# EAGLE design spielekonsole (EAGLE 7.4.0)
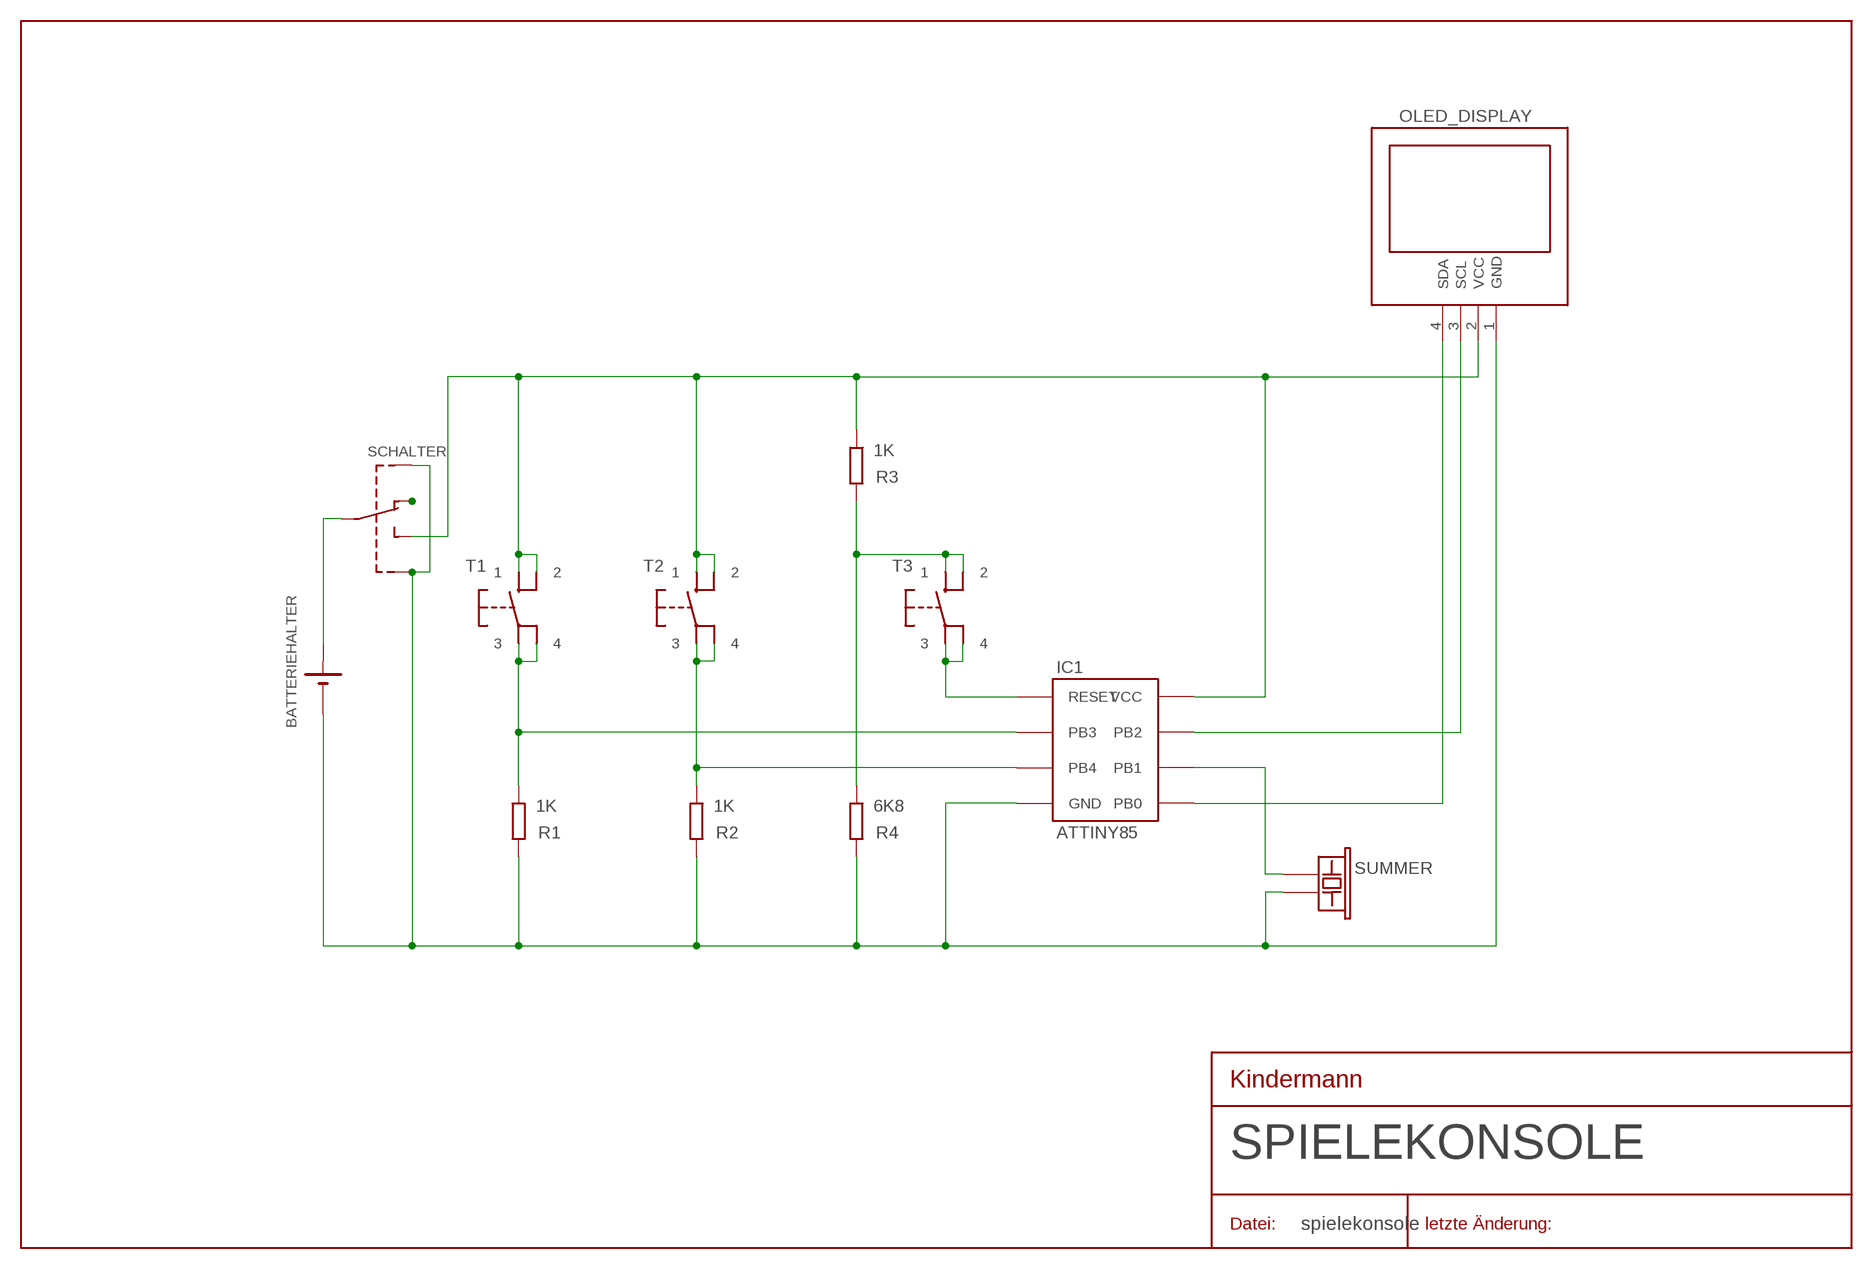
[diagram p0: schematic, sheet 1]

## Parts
BATTERIEHALTER  BATTERIEHALTER  [BATTERIEHALTER]
IC1  ATTINY85  [ATTINY85]
OLED_DISPLAY  OLED_DISPLAY  [OLED_DISPLAY]
R1  1K  WID-1K  [WID-1K]
R2  1K  WID-1K  [WID-1K]
R3  1K  WID-1K  [WID-1K]
R4  6K8  WID-6K8  [WID-6K8]
SCHALTER  S1  SCHIEBESCHALTER  [SCHIEBESCHALTER]
SUMMER  SUMMER  [SUMMER]
T1  MICROTASTER  [MICROTASTER]
T2  MICROTASTER  [MICROTASTER]
T3  MICROTASTER  [MICROTASTER]

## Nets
GND: BATTERIEHALTER.2(-) IC1.4(GND) OLED_DISPLAY.1(GND) R1.2 R2.2 R4.2 SCHALTER.4 SCHALTER.5 SUMMER.2
N$3: BATTERIEHALTER.1(+) SCHALTER.2
N$4: R3.2 R4.1 T3.1 T3.2
N$6: IC1.6(PB1) SUMMER.1
N$9: IC1.1(RESET) T3.3 T3.4
PB3: IC1.2(PB3) R1.1 T1.3 T1.4
PB4: IC1.3(PB4) R2.1 T2.3 T2.4
SCL: IC1.7(PB2) OLED_DISPLAY.3(SCL)
SDA: IC1.5(PB0) OLED_DISPLAY.4(SDA)
SW1_3: SCHALTER.3
VCC: IC1.8(VCC) OLED_DISPLAY.2(VCC) R3.1 SCHALTER.1 T1.1 T1.2 T2.1 T2.2

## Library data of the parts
BATTERIEHALTER = Spielekonsole:BATTERIEHALTER
IC1 = Spielekonsole:ATTINY85
OLED_DISPLAY = Spielekonsole:OLED_DISPLAY
R1-R3 = Spielekonsole:WID-1K
R4 = Spielekonsole:WID-6K8
SCHALTER = Spielekonsole:SCHIEBESCHALTER
SUMMER = Spielekonsole:SUMMER
T1-T3 = Spielekonsole:MICROTASTER

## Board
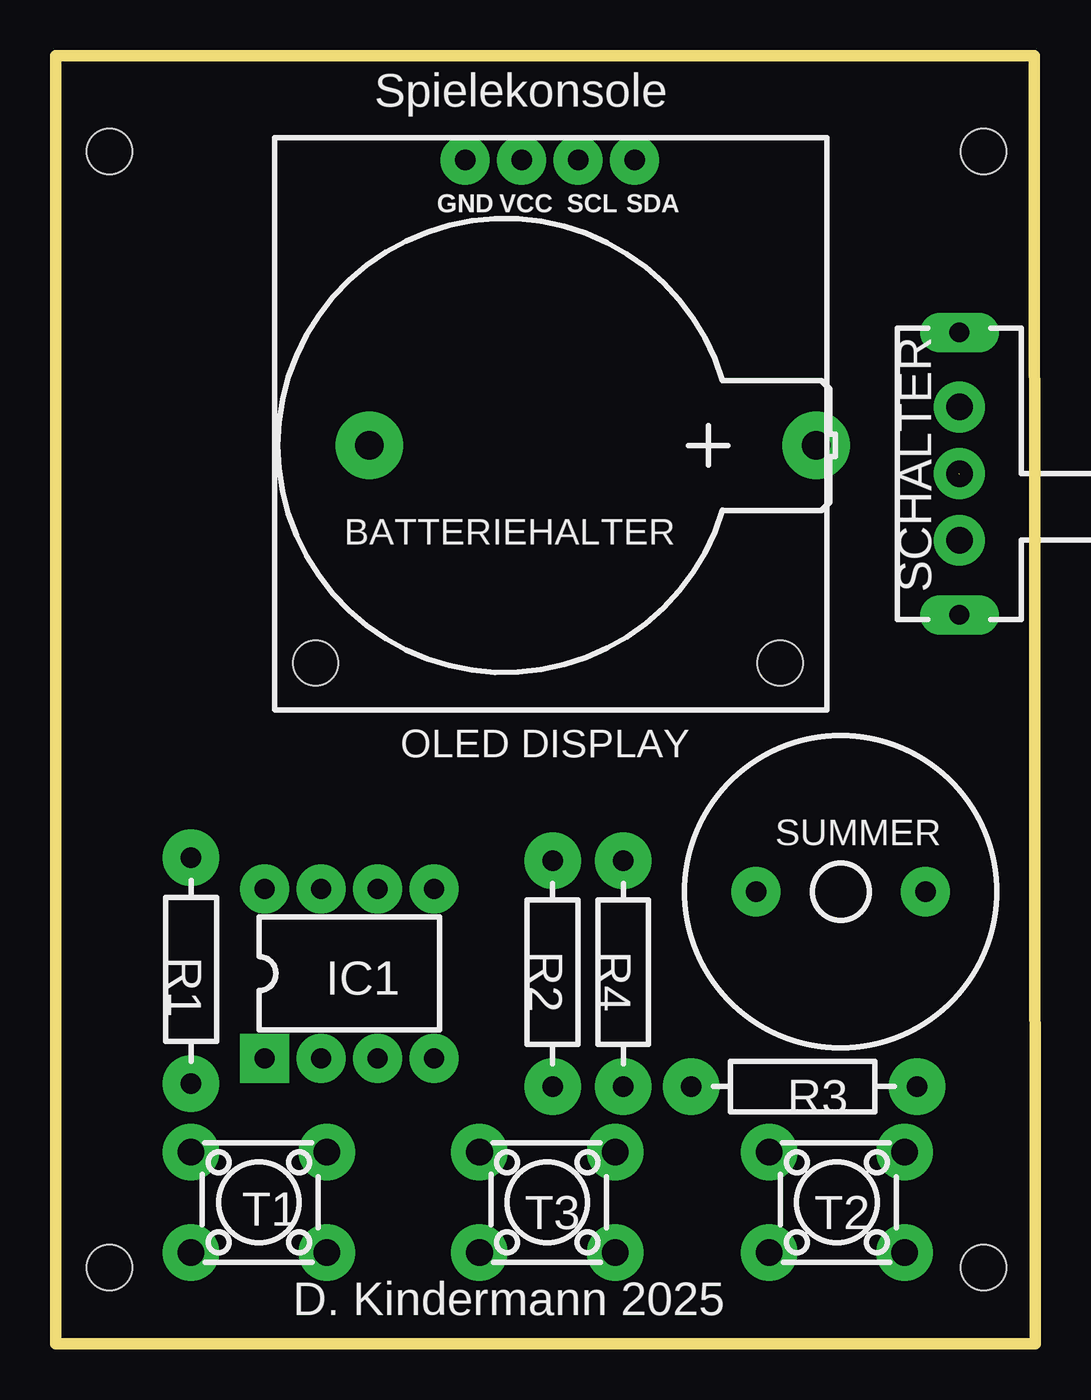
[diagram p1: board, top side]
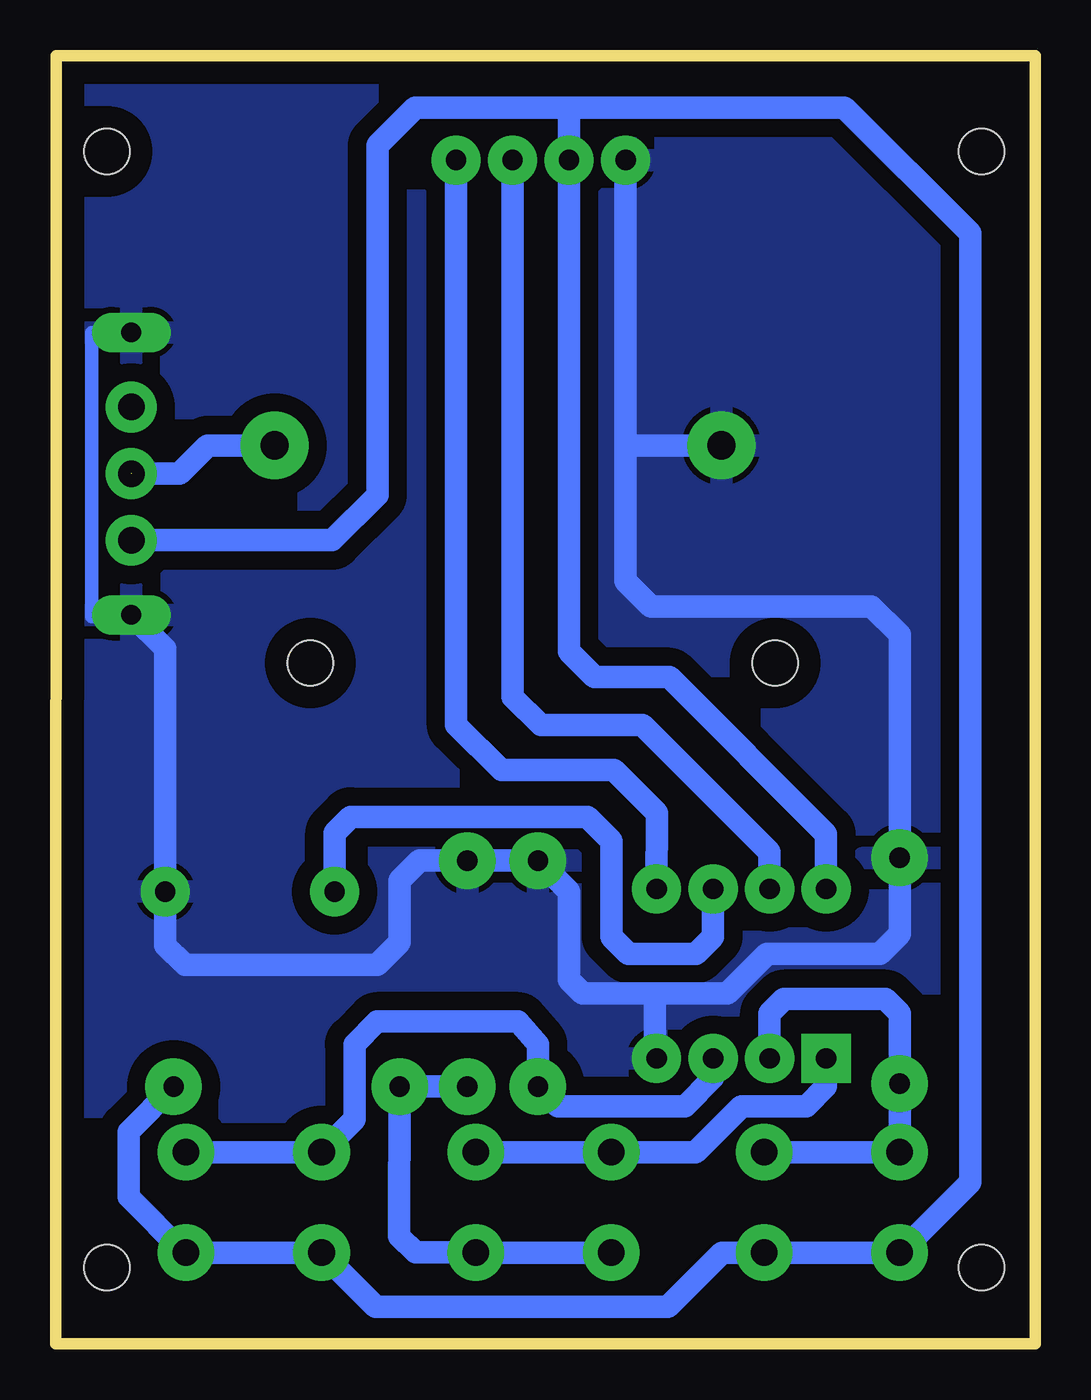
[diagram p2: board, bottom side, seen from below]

Size 44.04 x 57.92 mm. Coordinates in mm from the lower left corner, seen from the top.
Outline: 0,0.01 44.04,0 44.01,57.91 0,57.92 0,0.01
Copper layers (1*16): Top 0.035mm / dielectric 1.5mm / Bottom 0.035mm
Design rules "PCB-Spielekonsole_2025-05-16": minimum track width 10mil, minimum drill 24mil, track to track 8mil, track to pad 8mil, pad to pad 8mil, via to via 8mil, smd to smd 8mil, copper to edge 40mil, drill to drill 8mil, minimum pad ring 0mil, minimum via ring 0mil, stop-mask expansion 4mil, vias tented up to drill 0mil, thermal gap 10mil
Holes 2.03 mm at 2.41,53.61 41.73,53.61 11.69,30.61 32.58,30.61 2.41,3.44 41.73,3.44

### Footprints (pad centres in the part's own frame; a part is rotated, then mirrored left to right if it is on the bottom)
BATTERIEHALTER = drill 1.27 pad 3.048: 1 20.091,0; 2 0,0
ATTINY85 = drill 0.914 pad 2.21 square: 1 -3.81,3.81 | drill 0.914 pad 2.21: 2 -3.81,1.27; 3 -3.81,-1.27; 4 -3.81,-3.81; 5 3.81,-3.81; 6 3.81,-1.27; 7 3.81,1.27; 8 3.81,3.81
OLED_DISPLAY = drill 0.914 pad 2.21: 1 -3.81,0; 2 -1.27,0; 3 1.27,0; 4 3.81,0
WID-1K = drill 0.914 pad 2.54: 1 5.08,0; 2 -5.08,0
WID-6K8 = drill 0.914 pad 2.54: 1 5.08,0; 2 -5.08,0
SCHIEBESCHALTER = drill 1.194 pad 2.286: 1 -2.997,0; 2 0,0; 3 2.997,0 | drill 0.889 pad 1.778 long: 4 6.35,0; 5 -6.35,0
SUMMER = drill 0.914 pad 2.21: 1 3.81,0; 2 -3.81,0
MICROTASTER = drill 1.194 pad 2.54: 1 -3.048,2.261; 2 3.048,2.261; 3 -3.048,-2.261; 4 3.048,-2.261

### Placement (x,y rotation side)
BATTERIEHALTER  14.11,40.4 0 top
IC1  13.21,16.65 90 top
OLED_DISPLAY  22.22,53.23 0 top
R1  6.09,16.78 270 top
R2  22.35,16.65 270 top
R3  33.66,11.57 0 top
R4  25.53,16.65 270 top
SCHALTER  40.64,39.13 90 top
SUMMER  35.31,20.33 180 top
T1  9.14,6.36 180 top
T2  35.13,6.36 180 top
T3  22.11,6.36 180 top

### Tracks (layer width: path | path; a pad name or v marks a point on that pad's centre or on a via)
GND
  Bottom 0.61: SCHALTER.4 42.41,45.48 42.41,32.72 40.64,32.72 SCHALTER.5
  Bottom 1.016: 17.08,15.76 13.84,15.76 12.07,17.54 6.98,17.54 6.09,18.43 R1.2 | IC1.4 17.08,12.9 17.08,15.76 | 17.08,15.76 20.34,15.76 20.95,16.37 | 18.41,40.4 OLED_DISPLAY.1 18.38,53.31 | 18.41,40.4 18.41,34.3 17.27,33.16 7.36,33.16 6.09,31.89 R1.2 | BATTERIEHALTER.2 18.41,40.4 | 6.09,22.56 R1.2 | 20.95,16.4 20.95,20.33 R2.2 R4.2 27.69,21.73 28.57,20.84 28.57,18.05 29.59,17.03 38.23,17.03 39.12,17.92 SUMMER.2 39.12,31.25 SCHALTER.5
  pour Bottom (isolate 0.813): 0.13,57.92 44.07,57.92 44.07,0.01 0.13,0.01
N$3  (1 unrouted)
  Bottom 1.016: BATTERIEHALTER.1 37.21,40.4 38.48,39.13 40.62,39.13
N$4
  Bottom 1.016: R4.1 R3.2 28.59,4.84 27.85,4.11 T3.1 T3.2
N$6
  Bottom 1.016: IC1.6 14.48,18.3 15.24,17.54 18.29,17.54 19.05,18.3 19.05,22.62 20.13,23.7 30.78,23.7 31.5,22.98 SUMMER.1
N$9
  Bottom 1.016: IC1.1 9.4,11.57 10.29,10.68 13.21,10.68 15.28,8.61 T3.4 T3.3
PB3
  Bottom 1.016: IC1.2 11.94,14.87 11.3,15.51 6.73,15.51 6.09,14.87 R1.1 T1.4 T1.3
PB4
  Bottom 1.016: IC1.3 14.48,11.95 15.75,10.68 21.46,10.68 R2.1 22.35,13.47 23.24,14.49 29.59,14.49 30.61,13.47 30.61,10.11 T2.4 T2.3
SCL
  Bottom 1.016: OLED_DISPLAY.3 23.49,29.1 22.22,27.83 17.65,27.83 11.94,22.11 IC1.7
SDA
  Bottom 1.016: IC1.5 17,23.86 18.94,25.79 24,25.79 26.04,27.83 OLED_DISPLAY.4
VCC
  Bottom 0.813: T2.1 38.25,4.1
  Bottom 1.016: T2.1 T2.2 29.64,1.66 16.51,1.66 14.07,4.1 T1.1 T1.2 2.92,7.27 2.92,49.94 8.58,55.59 21.22,55.59 | IC1.8 9.4,22.94 16.45,29.98 19.81,29.98 20.95,31.13 OLED_DISPLAY.2 20.95,55.32 21.22,55.59 | SCHALTER.1 31.6,36.13 29.57,38.16 29.57,53.89 27.88,55.59 21.22,55.59 | 38.25,4.1 40.77,6.62 40.77,9.54 R3.1

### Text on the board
tPlace: Spielekonsole | D. Kindermann 2025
